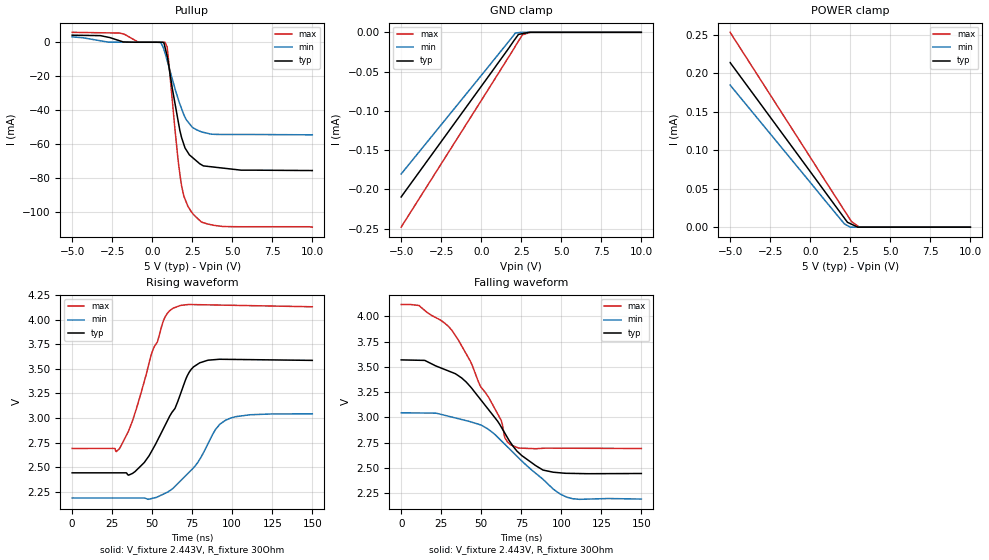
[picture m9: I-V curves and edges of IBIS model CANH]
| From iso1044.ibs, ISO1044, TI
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|   CANH
[Model]   CANH
Model_type   I/O_open_source
Polarity   Inverting
Enable   Active-Low
Vinl = 0.5
Vinh = 0.9
Vmeas = 3
Vref = 2.443
Cref = 2pF
Rref = 30
|   typ   min   max
C_comp   12.2e-12   11.49e-12   12.57e-12
[Voltage Range]   5   4.5   5.5
[Temperature Range]   25   150   -55
[Pullup Reference]   5   4.5   5.5
[Pulldown Reference]   0   0   0
[Power Clamp Reference]   5   4.5   5.5
[GND Clamp Reference]   0   0   0
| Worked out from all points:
|   slope of the pullup table from 0 to 0.75 V, typ, clamps not added: 727 ohm
|   falling waveform, V_fixture 2.443V, R_fixture 30Ohm: 20-80 % time 31.2ns typ, 35.1ns min, 29.3ns max; typ from 3.57 V to 2.44 V
|   rising waveform, V_fixture 2.443V, R_fixture 30Ohm: 20-80 % time 20.2ns typ, 21.6ns min, 16.6ns max; typ from 2.44 V to 3.59 V
[GND Clamp]
|   Voltage   I(typ)   I(min)   I(max)
-5V       -209.7uA   -180.5uA   -248.2uA
2.128V    -8.187uA   -910.9nA   -17.7uA
2.322V    -2.722uA   -432nA     -11.25uA
2.569V    -1.686uA   0A         -3.295uA
3.064V    0A         0A         0A
10V       0A         0A         0A
[Pullup]
|   Voltage   I(typ)   I(min)   I(max)
-5V       4.168mA    3.187mA    5.861mA
-2.061V   962.1uA    55.5uA     5.435mA
-861.1mV  8.134uA    7.958uA    128.5uA
482.5mV   3.073uA    -99.63uA   3.64uA
797.2mV   -2.85mA    -6.239mA   -7.214uA
930.8mV   -8.028mA   -10.68mA   -2.658mA
1.594V    -45.06mA   -32.61mA   -67.39mA
1.848V    -56.59mA   -39.51mA   -85.28mA
2.229V    -65.02mA   -46.88mA   -96.72mA
3.064V    -72.18mA   -52.81mA   -106mA
4.442V    -74.24mA   -54.38mA   -108.7mA
10V       -75.66mA   -54.59mA   -109mA
[POWER Clamp]
|   Voltage   I(typ)   I(min)   I(max)
-5V       213.6uA    184.5uA    252.9uA
2.128V    11.78uA    4.269uA    21.63uA
2.322V    6.298uA    2.025uA    15.35uA
2.569V    3.9uA      0A         7.37uA
3.064V    0A         0A         0A
10V       0A         0A         0A
[Ramp]
R_load = 30
|   typ   min   max
dV/dt_r   0.685442/2.00542e-08   0.512592/2.14191e-08   0.863536/1.66139e-08
dV/dt_f   0.674704/3.11586e-08   0.512317/3.5057e-08   0.855212/2.92131e-08
[Falling Waveform]
V_fixture = 2.443V
V_fixture_min = 2.188V
V_fixture_max = 2.691V
R_fixture = 30Ohm
C_fixture = 0F
|   Time   V(typ)   V(min)   V(max)
0s        3.569V     3.045V     4.117V
11.28ns   3.565V     3.043V     4.106V
31.67ns   3.445V     3.002V     3.861V
50.06ns   3.167V     2.923V     3.294V
62.3ns    2.909V     2.772V     2.975V
64.87ns   2.84V      2.731V     2.793V
68.51ns   2.745V     2.674V     2.726V
88.48ns   2.479V     2.388V     2.694V
103.4ns   2.446V     2.21V      2.694V
150ns     2.444V     2.191V     2.691V
[Rising Waveform]
V_fixture = 2.443V
V_fixture_min = 2.188V
V_fixture_max = 2.691V
R_fixture = 30Ohm
C_fixture = 0F
|   Time   V(typ)   V(min)   V(max)
0s        2.443V     2.188V     2.691V
29.42ns   2.443V     2.188V     2.686V
37.65ns   2.437V     2.188V     2.97V
45.02ns   2.548V     2.188V     3.371V
57.13ns   2.897V     2.228V     3.994V
62.96ns   3.071V     2.285V     4.115V
75.77ns   3.519V     2.493V     4.153V
89.67ns   3.594V     2.888V     4.148V
95.81ns   3.596V     2.978V     4.147V
150ns     3.586V     3.042V     4.13V
